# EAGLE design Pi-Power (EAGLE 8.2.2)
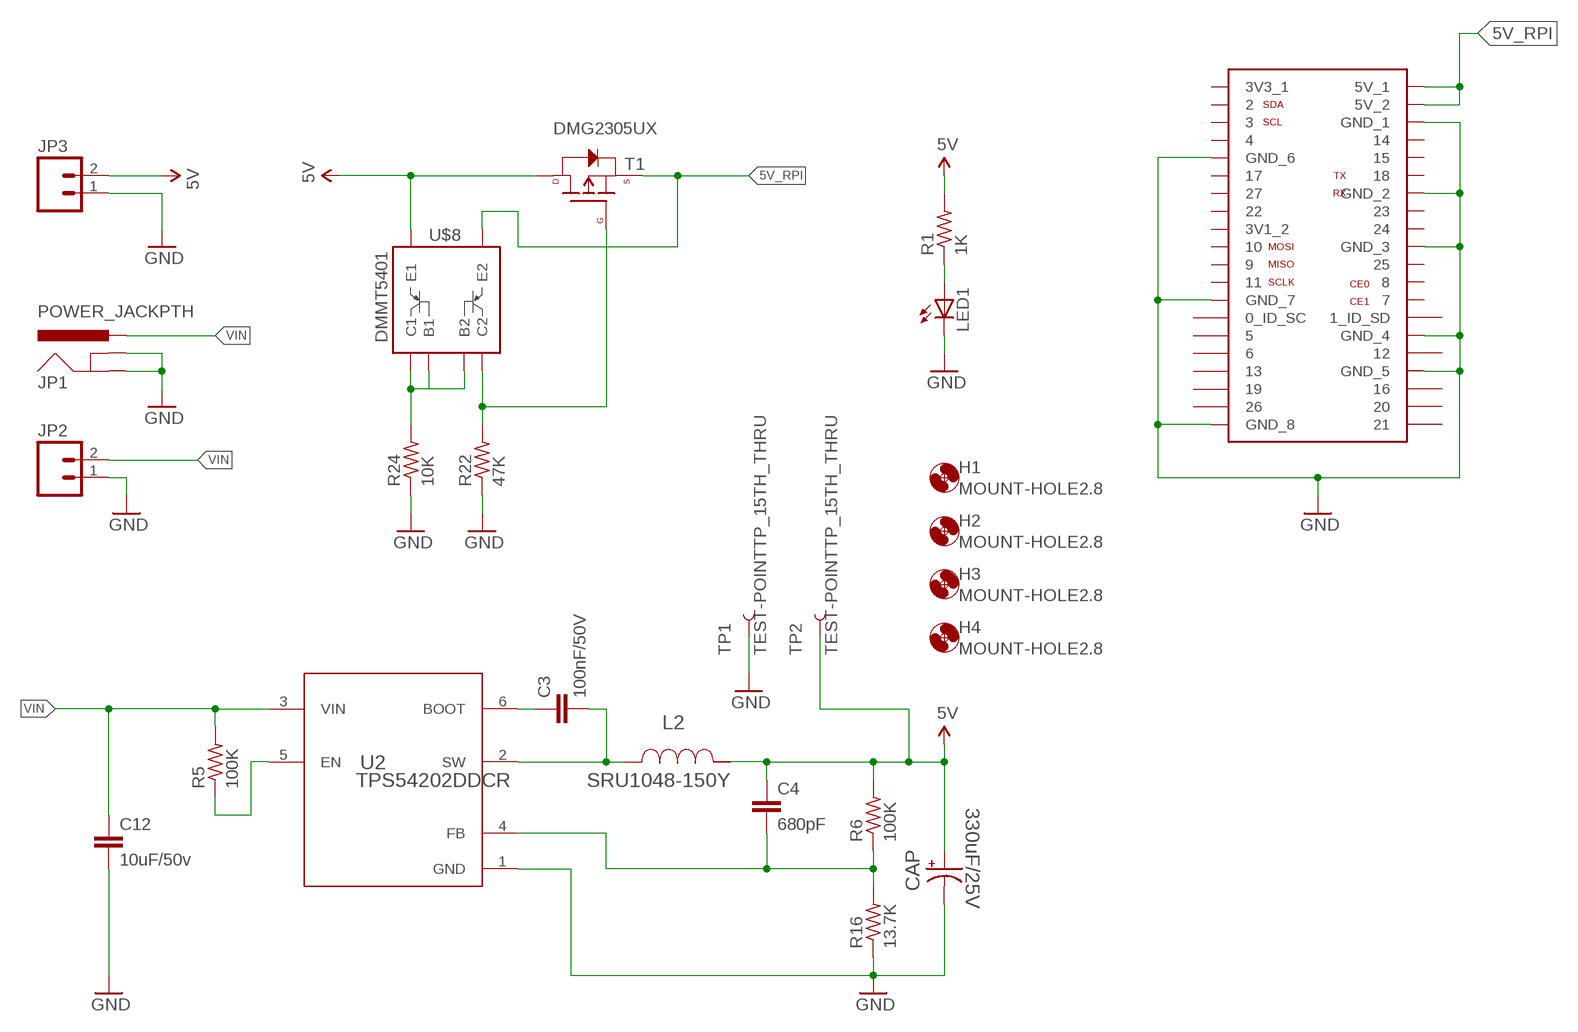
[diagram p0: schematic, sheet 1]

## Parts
C3  100nF/50V  CAP0805  [0805]
C4  680pF  CAP0603-CAP  [0603-CAP]
C12  10uF/50v  CAP1206  [1206]
CAP  330uF/25V  CAP_POLG  [PANASONIC_G]
H1  MOUNT-HOLE2.8  [2,8]
H2  MOUNT-HOLE2.8  [2,8]
H3  MOUNT-HOLE2.8  [2,8]
H4  MOUNT-HOLE2.8  [2,8]
JP1  POWER_JACKPTH  [POWER_JACK_PTH]
JP2  M025MM  [SCREWTERMINAL-5MM-2]
JP3  M02PTH  [1X02]
L2  SRU1048-150Y  [SRU1048]
LED1  LEDCHIPLED_0805  [CHIPLED_0805]
R1  1K  R-US_M0805  [M0805]
R5  100K  R-US_M0805  [M0805]
R6  100K  R-US_M0805  [M0805]
R16  13.7K  R-US_M0805  [M0805]
R22  47K  R-US_M0805  [M0805]
R24  10K  R-US_M0805  [M0805]
T1  DMG2305UX  P-CHANNEL-MOSFET  [SOT23-3]
TP1  TEST-POINTTP_15TH_THRU  [TP_15TH]
TP2  TEST-POINTTP_15TH_THRU  [TP_15TH]
U2  TPS54202DDCR  [DDC0006A_N]
U$1  RASPBERRY-PI-GPIO-SEPARATE  [2X20]
U$8  DMMT5401  [SOT-23-6]

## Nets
5V: C4.1 CAP.+ JP3.2 L2.2 R1.2 R6.2 T1.3(D) TP2.P$1 U$8.6(E1)
5V_RPI: T1.2(S) U$1.2(5V_1) U$1.4(5V_2) U$8.5(E2)
GND: C12.2 CAP.- JP1.GND JP1.GNDBREAK JP2.1 JP3.1 LED1.C R16.1 R22.1 R24.1 TP1.P$1 U2.1(GND) U$1.6(GND_1) U$1.9(GND_6) U$1.14(GND_2) U$1.20(GND_3) U$1.25(GND_7) U$1.30(GND_4) U$1.34(GND_5) U$1.39(GND_8)
N$1: LED1.A R1.1
N$2: R22.2 T1.1(G) U$8.4(C2)
N$5: R5.1 U2.5(EN)
N$7: C4.2 R6.1 R16.2 U2.4(FB)
N$18: C3.2 L2.1 U2.2(SW)
N$20: C3.1 U2.6(BOOT)
N$26: R24.2 U$8.1(C1) U$8.2(B1) U$8.3(B2)
VIN: C12.1 JP1.PWR JP2.2 R5.2 U2.3(VIN)
Unconnected: U$1.3 U$1.5 U$1.7 U$1.8 U$1.10 U$1.11 U$1.12 U$1.13 U$1.15 U$1.16 U$1.18 U$1.19 U$1.21 U$1.22 U$1.23 U$1.24 U$1.26 U$1.27(0_ID_SC) U$1.28(1_ID_SD) U$1.29 U$1.31 U$1.32 U$1.33 U$1.35 U$1.36 U$1.37 U$1.38 U$1.40

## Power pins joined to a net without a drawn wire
3V1_2: U$1.17(3V1_2)
3V3_1: U$1.1(3V3_1)

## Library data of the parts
C3 C12 = SparkFun-Capacitors:CAP: Capacitor
C4 = SparkFun-Passives:CAP: Capacitor
CAP = SparkFun-Passives:CAP_POL: Capacitor Polarized
H1-H4 = holes:MOUNT-HOLE: MOUNTING HOLE with drill center marker
JP1 = SparkFun-Connectors:POWER_JACK: Power Jack This is the standard 5.5mm barrel jack for power. The PTH is the most common, proven, reliable, footprint. The Slot footprint only works if the mill layer is transmitted to the PCB fab house so be warned. Mating wall wart : TOL-00298 (and others); PROD_ID: CONN-08197
JP2 = SparkFun-Connectors:M02: Standard 2-pin 0.1" header. Use with; STOREFRONT_ID: PRT-08432
JP3 = SparkFun-Connectors:M02: Standard 2-pin 0.1" header. Use with
L2 = AlainElements:SRU1048-150Y; DCR: 0.029; IDC: 3.2; L: 1.5E5; MANUFACTURER_NAME: Bourns; MANUFACTURER_PART_NUMBER: SRU1048150Y; VENDOR: Bourns
LED1 = adafruit:LED: LED
R1 R5 R6 R16 R22 R24 = resistor:R-US_: RESISTOR, American symbol
T1 = GeekAmmo:P-CHANNEL-MOSFET: P-Channel MOSFET Mode Field Effect Transistor
TP1 TP2 = SparkFun-Passives:TEST-POINT: Bare copper test points for troubleshooting or ICT
U2 = AlainElements:TPS54202DDCR; ALTERNATEPARTNUMBER: TPS54202DDCT; APPLICATION_BUILDNUMBER: *; COMPTYPE: IC; MANUFACTURER: Texas Instruments; MANUFACTURER_NAME: Texas Instruments; MANUFACTURER_PART_NUMBER: TPS54202DDCR; MOUNTTYPE: SMT; PACKAGEREFERENCE: DDC0006A; PARTNUMBER: TPS54202DDCR; PIN_COUNT: 6; REFDES: RefDes; ROHS: Y; TYPE: TYPE; VALUE: Value
U$1 = pimoroni-headers:RASPBERRY-PI-GPIO-SEPARATE
U$8 = pimoroni-ics:DMMT5401

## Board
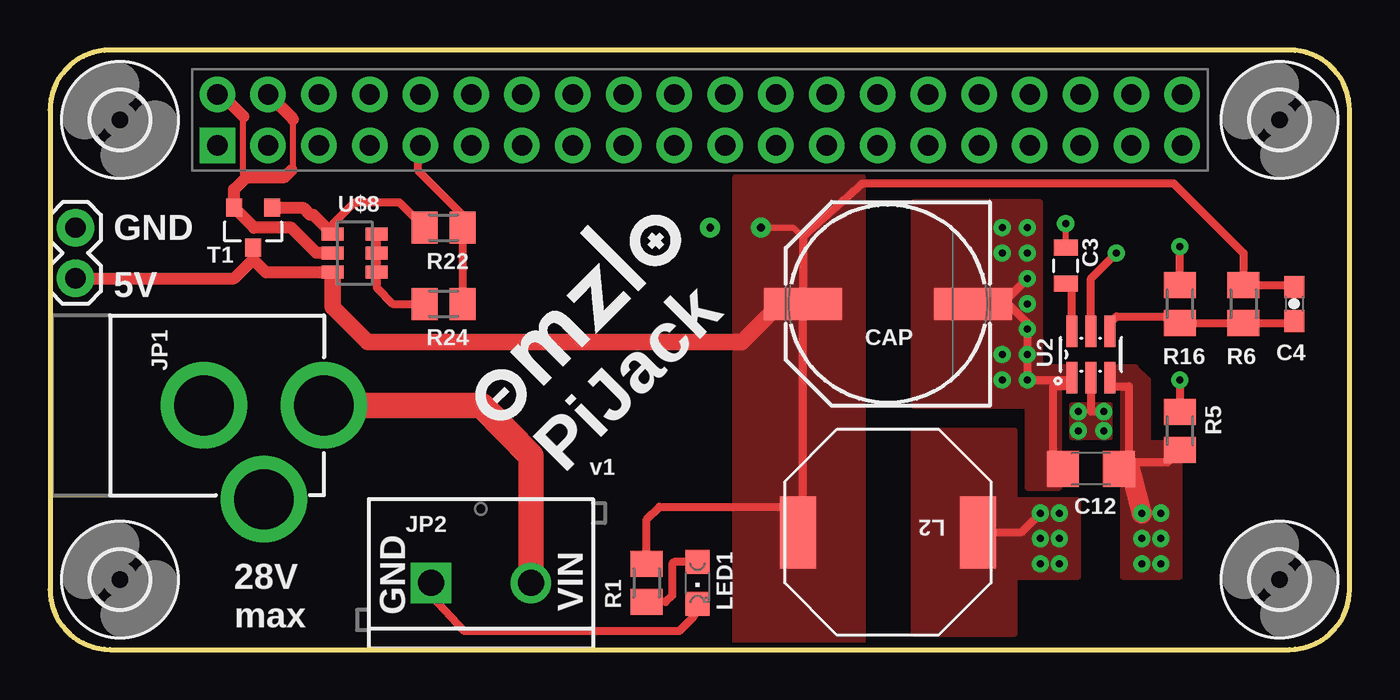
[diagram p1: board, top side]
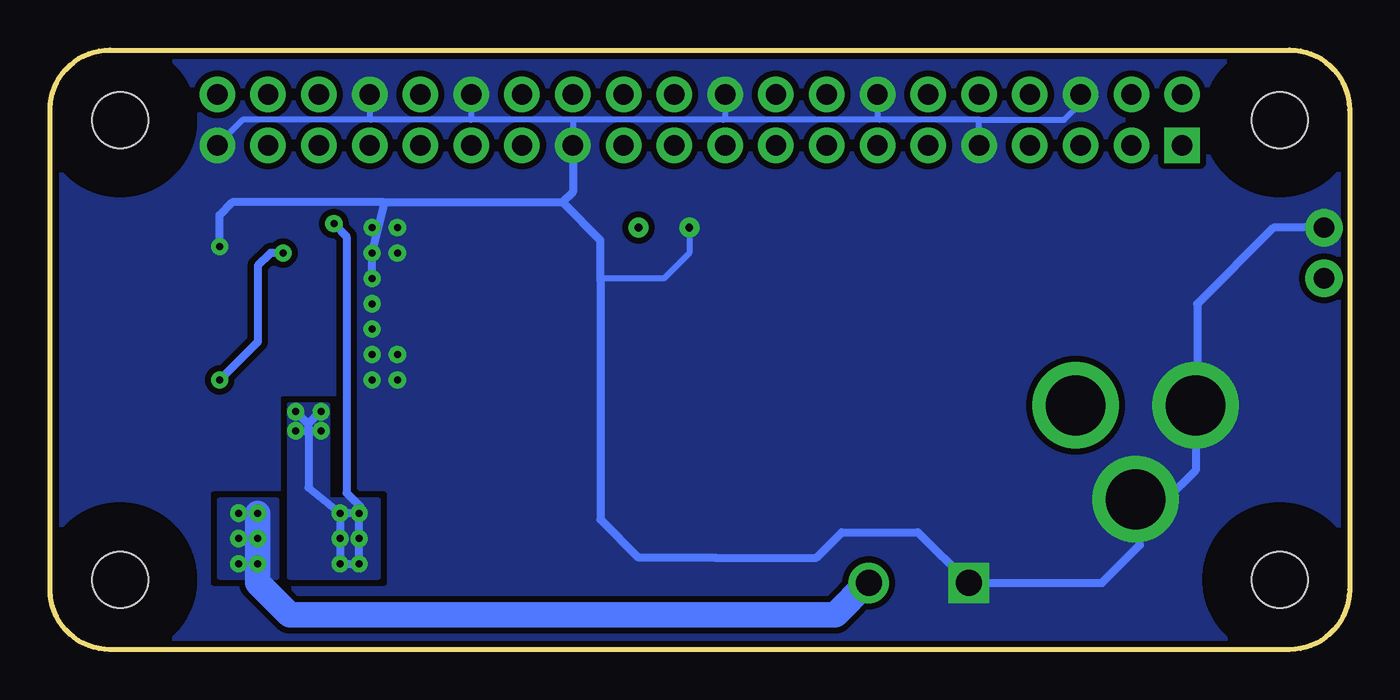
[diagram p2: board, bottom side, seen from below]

Size 65 x 30 mm. Coordinates in mm from the lower left corner, seen from the top.
Outline: 3,30 arc90 0,27 0,3 arc90 3,0 62,0 arc90 65,3 65,27 arc90 62,30 3,30
Copper layers (1*16): Top 0.035mm / dielectric 1.5mm / Bottom 0.035mm
Design rules "SparkFun": minimum track width 8mil, minimum drill 12mil, track to track 8mil, track to pad 8mil, pad to pad 8mil, via to via 8mil, smd to smd 8mil, copper to edge 10mil, drill to drill 8mil, minimum pad ring 12mil, minimum via ring 10mil, stop-mask expansion 4mil, vias tented up to drill 25mil, thermal gap 10mil

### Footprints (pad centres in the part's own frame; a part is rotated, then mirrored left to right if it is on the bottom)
0805 = smd 0.8 x 1.2: 1 -0.9,0; 2 0.9,0
0603-CAP = smd 1.1 x 1: 1 -0.85,0; 2 0.85,0
1206 = smd 1.6 x 1.8: 1 -1.4,0; 2 1.4,0
PANASONIC_G = smd 3.9 x 1.6: + 4.25,0; - -4.25,0
2,8 = hole 2.8: 0,0
POWER_JACK_PTH = drill 2.997 pad 4.318: GND 0,7.7; GNDBREAK 4.7,10.7; PWR 0,13.7
SCREWTERMINAL-5MM-2 = drill 1.3 pad 2.032 square: 1 0,0 | drill 1.3 pad 2.032: 2 5,0
1X02 = drill 1.016 pad 1.88: 1 0,0; 2 2.54,0
SRU1048 = smd 1.803 x 3.607: 1 -4.496,0; 2 4.496,0
CHIPLED_0805 = smd 1.2 x 1.2: A 0,-1.05; C 0,1.05
M0805 = smd 1.3 x 1.6: 1 -0.95,0; 2 0.95,0
SOT23-3 = smd 0.8 x 0.9: 1 -0.95,-1; 2 0.95,-1; 3 0,1
TP_15TH = drill 0.381 pad 0.61: P$1 0,0
DDC0006A_N = smd 1.575 x 0.559: 1 -1.168,0.95; 2 -1.168,0; 3 -1.168,-0.95; 4 1.168,-0.95; 5 1.168,0; 6 1.168,0.95
2X20 = drill 1.016 pad 1.778 square: 1 -24.13,-1.27 | drill 1.016 pad 1.778: 2 -24.13,1.27; 3 -21.59,-1.27; 4 -21.59,1.27; 5 -19.05,-1.27; 6 -19.05,1.27; 7 -16.51,-1.27; 8 -16.51,1.27; 9 -13.97,-1.27; 10 -13.97,1.27; 11 -11.43,-1.27; 12 -11.43,1.27; 13 -8.89,-1.27; 14 -8.89,1.27; 15 -6.35,-1.27; 16 -6.35,1.27; 17 -3.81,-1.27; 18 -3.81,1.27; 19 -1.27,-1.27; 20 -1.27,1.27; 21 1.27,-1.27; 22 1.27,1.27; 23 3.81,-1.27; 24 3.81,1.27; 25 6.35,-1.27; 26 6.35,1.27; 27 8.89,-1.27; 28 8.89,1.27; 29 11.43,-1.27; 30 11.43,1.27; 31 13.97,-1.27; 32 13.97,1.27; 33 16.51,-1.27; 34 16.51,1.27; 35 19.05,-1.27; 36 19.05,1.27; 37 21.59,-1.27; 38 21.59,1.27; 39 24.13,-1.27; 40 24.13,1.27
SOT-23-6 = smd 0.65 x 1.1: 1 0.95,1.1; 2 0,1.1; 3 -0.95,1.1; 4 -0.95,-1.1; 5 0,-1.1; 6 0.95,-1.1

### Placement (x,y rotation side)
C3  50.8,19.2 90 top
C4  62.23,17.3 270 top
C12  52.07,9.04 180 top
CAP  41.91,17.3 180 top
H1  3.5,26.5 270 top
H2  3.5,3.5 270 top
H3  61.5,26.5 270 top
H4  61.5,3.5 270 top
JP1  0,12.22 270 top
JP2  19.05,3.33 0 top
JP3  1.27,21.11 270 top
L2  41.91,5.87 180 top
LED1  32.38,3.33 180 top
R1  29.84,3.33 90 top
R5  56.52,10.95 270 top
R6  59.69,17.3 90 top
R16  56.52,17.3 270 top
R22  19.68,21.11 180 top
R24  19.68,17.3 180 top
T1  10.16,21.11 180 top
TP1  33.02,21.11 270 top
TP2  35.56,21.11 270 top
U2  52.07,14.76 90 top
U$1  32.5,26.5 0 top
U$2  [OMZLO-0.5]  22.54,10.95 45 top
U$8  15.24,19.84 270 top

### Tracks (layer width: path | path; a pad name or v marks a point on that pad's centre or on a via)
5V
  Top 0.305: TP2.P$1 37.19,21.11 37.66,20.63
  Top 0.406: 37.66,7.08 37.66,17.06 | 37.66,7.08 37.66,6.12 L2.2 | 37.66,17.06 CAP.+ 37.66,20.63 37.66,20.67 40.64,23.33 56.2,23.33 59.69,19.84 R6.2 62.13,18.25 C4.1 | 10.16,19.52 T1.3 | U$8.6 | 37.42,17.3 37.66,17.06 | 35.56,16.31 36.86,17.3 | R1.2 29.84,6.51 30.48,7.14 37.6,7.14 37.66,7.08
  Top 0.61: U$8.6 10.79,18.89 10.16,19.52 9.21,18.57 JP3.2 | 14.14,18.46 U$8.6
  Top 0.813: 37.42,17.3 36.86,17.3 36.51,17.3 34.61,15.39 19.68,15.39 15.88,15.39 14.14,17.13 14.14,18.46
  pour Top (no thermals): 34.29,-0.16 34.29,23.65 40.64,23.65 40.64,-0.16
5V_RPI
  Top 0.305: 9.84,23.59 9.66,23.76 9.66,26.68 | 12.15,24.08 12.15,26.52
  Top 0.406: U$1.2 8.37,27.66 | 9.84,23.65 9.84,23.59 | 12.06,23.97 12.06,23.99 12.15,24.08
  Top 0.61: U$8.5 13.34,19.84 12.06,21.11 10.21,21.11 T1.2 9.21,23.02 9.84,23.65 11.75,23.65 12.06,23.97 | 9.66,26.68 8.69,27.66 8.37,27.66 | 12.15,26.52 U$1.4
GND  (via drill 0.35)
  Top 0.406: U2.1 51.12,13.17 50.16,13.17 50.16,9.04 C12.2 | U2.1 | U2.1 51.02,13.49 49.21,13.49 48.9,13.81 48.9,16.35 47.94,17.3 47.62,17.3 | R16.1 v56.52,20.16 | CAP.- 47.62,17.3 | 47.62,17.3 v48.9,18.57 | U$1.9 18.41,25.11 18.41,23.97 20.64,21.75 R22.1 R24.1 | JP2.1 19.05,2.69 20.72,0.93 31.47,0.93 32.19,1.65 LED1.C
  Bottom 0.305: U$1.6 13.45,27.34 14.29,26.51 18.5,26.51 | 43.95,26.51 48.94,26.51 | 38.81,26.51 43.95,26.51 | 31.32,26.51 38.81,26.51 | 23.51,26.51 31.32,26.51 | 18.5,26.51 23.51,26.51 | 48.94,26.51 55.35,26.51 U$1.39 | U$1.34 49.01,26.58 48.94,26.51 | U$1.30 43.93,26.53 43.95,26.51 | U$1.25 38.85,26.47 38.81,26.51 | U$1.20 31.23,26.6 31.32,26.51 | U$1.14 23.61,26.61 23.51,26.51 | U$1.9 18.53,26.48 18.5,26.51 | 31.75,4.62 31.73,4.6 | TP1.P$1 33.02,19.84 34.29,18.57 37.36,18.57 37.47,18.47
  Bottom 0.406: v56.52,20.16 56.52,21.75 55.88,22.38 48.31,22.38 | 48.31,22.38 39.37,22.38 | 39.37,22.38 37.47,20.47 37.47,18.47 37.47,6.51 35.56,4.6 31.73,4.6 26.67,4.6 25.4,5.87 21.59,5.87 JP2.1 12.38,3.33 10.48,5.23 10.48,7.3 JP1.GNDBREAK 10.64,7.46 9.21,7.46 7.7,8.96 JP1.GND 7.62,12.3 7.62,17.3 3.81,21.11 JP3.1 | U$1.25 38.85,22.9 39.37,22.38 | v48.9,18.57 v48.9,19.84 48.26,22.33 48.31,22.38
  other vias: 47.62,21.11 48.9,21.11 47.62,19.84 48.9,16.03 47.62,14.76 48.9,14.76 48.9,13.49 47.62,13.49 48.9,17.3
  pour Bottom (isolate 0.305, rank 2, no thermals): 66.04,30 0,30 0,-0.48 66.04,-0.48
  pour Top (no thermals): 43.18,22.38 43.18,12.22 48.9,12.22 48.9,8.09 50.48,8.09 50.48,13.17 51.12,13.17 51.12,14.12 49.53,14.12 49.53,22.38
N$1
  Top 0.406: LED1.A 31.21,4.38 31.11,4.28 31.11,2.69 30.8,2.38 R1.1
N$2
  Top 0.406: 13.02,21.75 13.19,21.75 | U$8.4 14.14,21.28 15.24,22.38 17.46,22.38 R22.2
  Top 0.61: T1.1 12.65,22.11 13.02,21.75 | 13.19,21.75 U$8.4
N$5  (via drill 0.35)
  Top 0.406: U2.5 52.07,18.57 v53.34,19.84 | v56.52,13.49 R5.1
  Bottom 0.406: v53.34,19.84 53.98,19.84 54.61,19.2 54.61,15.39 v56.52,13.49
N$7
  Top 0.406: U2.4 53.02,16.34 53.34,16.66 56.2,16.66 56.45,16.41 R16.2 R6.1 62.13,16.35 C4.2
N$18  (via drill 0.35)
  Top 0.305: C3.2 v50.8,21.31
  Top 0.406: U2.2 52.07,11.9 v52.7,11.9 | L2.1 48.58,5.87 v49.53,6.82
  Bottom 0.406: 52.07,10.95 52.07,8.09 v50.48,6.82 | 49.48,7.14 v49.53,6.82 v50.48,6.82 | v50.8,21.31 50.16,20.68 50.16,7.83 49.48,7.14 | 52.1,11.29 52.07,10.95 | 52.1,11.29 v52.7,11.9 | v51.44,11.9 51.49,11.9 52.1,11.29 | v50.48,6.82 v50.48,5.55 v50.48,4.28 v49.53,4.28 v49.53,5.55 49.53,7.09 49.48,7.14 | v51.44,10.95 52.07,10.95 | v52.7,10.95 52.07,10.95
  pour Top (no thermals): 51.44,7.46 48.26,7.46 48.26,10.95 43.18,10.95 43.18,0.79 48.26,0.79 48.26,3.65 51.44,3.65
  pour Top (isolate 0.305): 53.02,12.22 51.12,12.22 51.12,10.63 53.02,10.63
  pour Bottom (isolate 0.305): 53.02,12.22 53.02,3.65 48.58,3.65 48.58,7.46 51.12,7.46 51.12,12.22
N$20
  Top 0.406: U2.6 51.12,17.98 C3.1
N$26
  Top 0.406: U$8.3 U$8.2 U$8.1 16.34,18.11 17.14,17.3 R24.2
VIN  (via drill 0.35)
  Top 0.406: U2.3 53.02,13.17 53.98,13.17 53.98,9.2 | 53.98,9.2 53.98,9.04 C12.1 | R5.2 55.88,9.36 54.14,9.36 53.98,9.2 | JP1.PWR 13.97,12.22
  Top 1.016: v54.61,6.82 53.98,9.2
  Top 1.27: 13.97,12.22 21.59,12.22 24.05,9.68 JP2.2
  Bottom 0.406: JP2.2 24.13,3.33
  Bottom 1.27: 24.13,3.33 25.72,1.74 53.02,1.74 54.61,3.33 v54.61,4.28 v54.61,5.55 v54.61,6.82
  other vias: 55.56,4.28 55.56,5.55 55.56,6.82
  pour Top (isolate 0.305, no thermals): 53.02,14.12 53.02,13.17 53.66,13.17 53.66,3.65 56.52,3.65 56.52,10.31 54.93,10.31 54.93,13.49 54.29,14.12
  pour Bottom: 53.66,3.65 53.66,7.46 56.52,7.46 56.52,3.65

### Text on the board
tNames: GND | 5V | PiJack | v1 | VIN | 28V / max | GND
